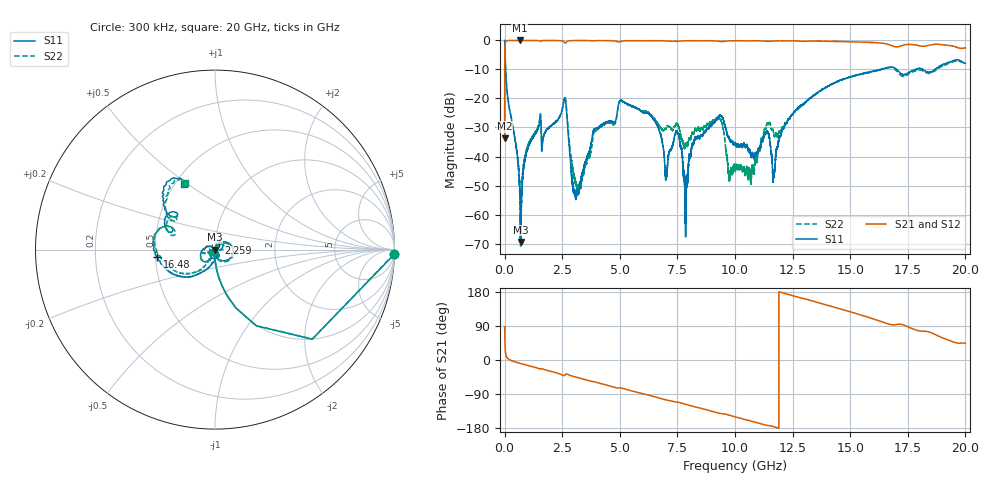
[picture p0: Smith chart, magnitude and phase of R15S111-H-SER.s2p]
!{R15S111}
!Johanson Technology Inc.
!www.johansontechnology.com
!Test Board Conditions:
!Substrate Type  RO4350B
!Substrate Thickness  20 mil
!Substrate Dk  3.66
!TL Type: GCPW
!TL Trace Width  34 mil
!TL Gap  10 mil
!Electrode orientation  Horizontal
!DUT TOPOLOGY	SERIES
!Mounting Pad LxW  26x52 mil
! Created Sat Feb  6 14:08:07 2021
# hz S ma R 50
! 2 Port Network Data from SP1.SP block
! freq  magS11  angS11  magS21  angS21  magS12  angS12  magS22  angS22
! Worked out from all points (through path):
!   20001 points, 300 kHz to 20 GHz, reference 50 ohm
!   highest |S21| = 0.00 dB at 648.3 MHz (marker M1); lowest = -33.7 dB at 300 kHz (marker M2)
!   group delay of S21, straight-line fit = 44.2 ps
!   lowest |S11| = -69.4 dB at 704.3 MHz (marker M3), VSWR 1.00, Z = 50 - j0.0176 ohm
!   |S11| at or under -10 dB: 43.25 MHz to 16.35 GHz (16.31 GHz wide, 199 % of centre); 17.02 GHz to 17.82 GHz (804.6 MHz wide, 4.62 % of centre); 18.15 GHz to 18.68 GHz (536.2 MHz wide, 2.91 % of centre)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
!   |S22| runs from -70.9 to 0.0 dB; largest |S21 - S12| = 0.018
!   S11 on the Smith chart (normalised r, x): 300 kHz: 1, -78; 2.259 GHz: 1.04, +0.07; 16.48 GHz: 0.51, -0.04; 20 GHz: 0.56, +0.48
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300000  0.9998 -1.5  0.02072 87.9  0.02079 88.4  0.9981 -1.4
1.093e8  0.1299 -84.0  0.9911 5.9  0.9912 5.9  0.1305 -84.1
6.483e8  0.003543 -104.0  0.9999 -8.5  0.9986 -8.4  0.002969 -103.2
7.043e8  0.0003387 -148.7  0.9996 -9.4  0.9988 -9.4  0.001023 113.4
1.4783e9  0.03255 68.9  0.9961 -22.3  0.996 -22.3  0.03463 61.6
2.2593e9  0.04145 60.1  0.9957 -34.1  0.9957 -34.1  0.04055 46.3
2.6203e9  0.1033 -14.1  0.9011 -39.9  0.9014 -39.9  0.1069 -17.7
3.0103e9  0.002502 -44.1  0.9954 -43.8  0.9951 -43.8  0.004636 -62.4
3.3343e9  0.003993 -92.4  0.9966 -49.2  0.9962 -49.1  0.003729 -127.5
5.0433e9  0.09375 -143.1  0.9598 -73.6  0.9611 -73.6  0.09296 -144.8
6.6673e9  0.03191 147.0  0.9905 -99.6  0.9905 -99.6  0.03607 -152.1
7.0183e9  0.004445 -155.2  0.9783 -105.4  0.9789 -105.4  0.03115 -119.4
7.5103e9  0.02592 -149.3  0.9671 -111.4  0.9665 -111.4  0.03634 -124.0
7.8603e9  0.001438 13.3  0.9879 -116.9  0.9884 -116.9  0.01617 -87.9
9.3073e9  0.04919 -86.7  0.9684 -140.5  0.9682 -140.4  0.04623 -77.3
1.00003e10  0.01746 -126.9  0.987 -149.9  0.987 -149.9  0.006556 -39.2
1.13883e10  0.02677 -127.0  0.9648 -172.6  0.9663 -172.6  0.03728 -155.7
1.16833e10  0.004692 -93.7  0.9787 -176.0  0.9787 -176.0  0.02482 -172.3
1.33343e10  0.1062 -109.3  0.9774 156.3  0.9785 156.2  0.1056 -121.6
1.64783e10  0.3251 -173.1  0.8851 98.5  0.8772 98.7  0.33 179.0
1.66673e10  0.3406 177.9  0.8528 94.7  0.8368 94.8  0.3457 171.9
2e10  0.4017 115.5  0.7489 44.3  0.7426 44.1  0.4059 114.3
